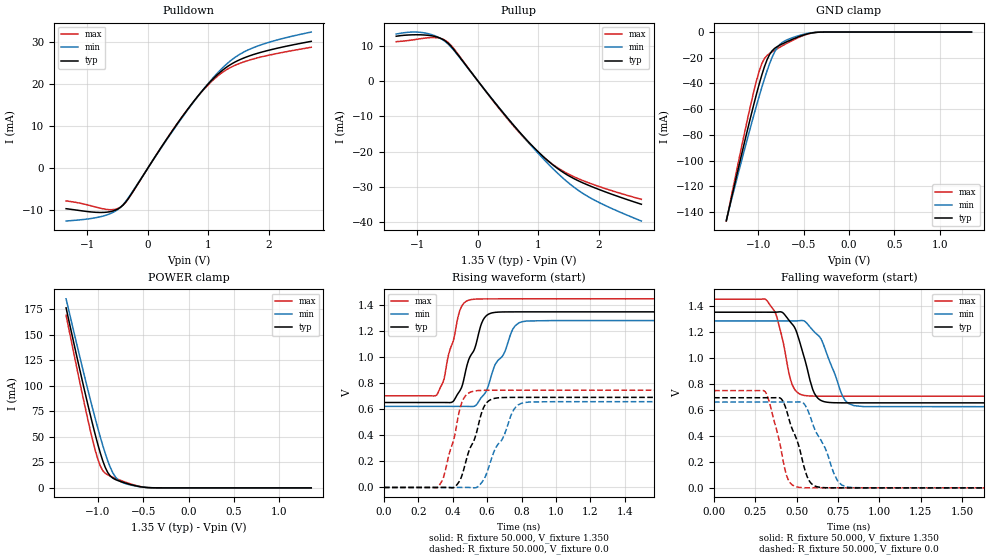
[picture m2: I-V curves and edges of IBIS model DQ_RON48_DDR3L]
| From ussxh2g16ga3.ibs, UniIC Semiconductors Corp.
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|   Model DQ_RON48_DDR3L
[Model] DQ_RON48_DDR3L
Model_type I/O
Vinl =  0.540V
Vinh =  0.810V
Vmeas =  0.675V
Rref =  50.000
Vref =  0.675V
C_comp   0.966pF   0.965pF   0.967pF
[Model Spec]
Vinh   0.810V   0.776V   0.860V
Vinl   0.540V   0.506V   0.590V
Vmeas   0.675V   0.641V   0.725V
Vref   0.675V   0.641V   0.725V
Rref   50.000   NA   NA
[Temperature Range]   25.000   95.000   -40.000
[Voltage Range]   1.350V   1.283V   1.450V
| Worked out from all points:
|   slope of the pulldown table from 0 to 0.203 V, typ, clamps not added: 44.6 ohm
|   slope of the pullup table from 0 to 0.203 V, typ, clamps not added: 45.5 ohm
|   GND clamp passes 1 mA (typ) near -0.43 V on its own axis
|   POWER clamp passes 1 mA (typ) near -0.52 V on its own axis
|   rising waveform, R_fixture 50.000, V_fixture 1.350: 20-80 % time 98.5ps typ, 130ps min, 76.3ps max; typ from 0.653 V to 1.35 V
|   rising waveform, R_fixture 50.000, V_fixture 0.0: 20-80 % time 99.3ps typ, 128ps min, 79.9ps max; typ from 0 V to 0.693 V
|   falling waveform, R_fixture 50.000, V_fixture 1.350: 20-80 % time 93.1ps typ, 118ps min, 75.9ps max; typ from 1.35 V to 0.653 V
|   falling waveform, R_fixture 50.000, V_fixture 0.0: 20-80 % time 102ps typ, 132ps min, 80.6ps max; typ from 0.693 V to 0 V
[Pulldown]
|Voltage   I(typ)   I(min)   I(max)
-1.35V    -9.661mA   -12.6mA    -7.804mA
-735mV    -10.55mA   -11.4mA    -9.699mA
-571mV    -10.19mA   -10.52mA   -9.878mA
-448mV    -9.296mA   -9.283mA   -9.257mA
-325mV    -7.31mA    -7.136mA   -7.371mA
249mV     5.557mA    5.434mA    5.606mA
618mV     13.25mA    13.09mA    13.27mA
905mV     18.55mA    18.56mA    18.43mA
1.151V    22.32mA    22.69mA    21.94mA
1.397V    24.97mA    25.97mA    24.24mA
1.684V    26.81mA    28.38mA    25.8mA
2.7V      30.25mA    32.47mA    28.84mA
[Pullup]
|Voltage   I(typ)   I(min)   I(max)
-1.35V    12.67mA    13.29mA    11.13mA
-908mV    13.04mA    13.68mA    12.07mA
-703mV    12.57mA    12.74mA    12.28mA
-539mV    11.33mA    11.14mA    11.5mA
-416mV    9.28mA     9.055mA    9.534mA
568mV     -12.09mA   -12.06mA   -12.31mA
855mV     -17.57mA   -17.78mA   -17.76mA
1.142V    -22.35mA   -23.11mA   -22.34mA
1.429V    -26.07mA   -27.83mA   -25.71mA
1.757V    -28.99mA   -32.05mA   -28.32mA
2.126V    -31.5mA    -35.4mA    -30.55mA
2.7V      -34.86mA   -39.6mA    -33.47mA
[GND_clamp]
|Voltage   I(typ)   I(min)   I(max)
-1.35V    -146.9mA   -146.3mA   -147.1mA
-1.126V   -78.8mA    -85.17mA   -70.77mA
-1.014V   -47.25mA   -56.31mA   -36.92mA
-958mV    -33.17mA   -42.77mA   -24.44mA
-930mV    -26.97mA   -36.36mA   -20.61mA
-874mV    -17.51mA   -24.69mA   -16.72mA
-818mV    -12.71mA   -15.46mA   -14.21mA
-762mV    -10.26mA   -9.751mA   -11.88mA
-706mV    -8.307mA   -6.907mA   -9.644mA
-538mV    -3.274mA   -2.499mA   -3.731mA
-398mV    -591.2uA   -439.3uA   -663.7uA
1.35V     0A         0A         0A
[POWER_clamp]
|Voltage   I(typ)   I(min)   I(max)
-1.35V    176.6mA    185.4mA    169.4mA
-1.198V   115.5mA    128.2mA    103.2mA
-1.114V   83.04mA    97.6mA     68.48mA
-1.058V   62.42mA    77.92mA    46.98mA
-1.002V   43.19mA    59.09mA    28.56mA
-946mV    26.54mA    41.57mA    16.92mA
-890mV    14.85mA    26.22mA    12.66mA
-834mV    9.439mA    14.55mA    10.39mA
-778mV    7.089mA    7.901mA    8.361mA
-638mV    3.198mA    2.764mA    3.815mA
-414mV    126.6uA    165.9uA    94.28uA
1.35V     0A         0A         0A
[Ramp]
| variable   typ   min   max
dV/dt_r   0.416/99.045p   0.396/0.128n   0.448/79.809p
dV/dt_f   0.418/92.332p   0.396/0.118n   0.447/75.961p
R_load = 50.000
[Rising Waveform]
R_fixture= 50.000
V_fixture= 1.350
V_fixture_min= 1.283
V_fixture_max= 1.450
|time   V(typ)   V(min)   V(max)
0s        653.2mV    623.3mV    704.3mV
306ps     653.2mV    623.3mV    710.5mV
348ps     653.2mV    623.3mV    827.3mV
406ps     667.2mV    623.3mV    1.141V
450ps     764.2mV    623.3mV    1.388V
507ps     1.02V      622.3mV    1.444V
598ps     1.323V     749.6mV    1.45V
751ps     1.35V      1.221V     1.45V
801ps     1.35V      1.274V     1.45V
3ns       1.35V      1.283V     1.45V
[Rising Waveform]
R_fixture= 50.000
V_fixture= 0.0
V_fixture_min= 0.0
V_fixture_max= 0.0
|time   V(typ)   V(min)   V(max)
0s        157.3nV    1.097uV    72.97nV
316ps     -25.78uV   3.116uV    5.409mV
348ps     124.4uV    5.006uV    85.1mV
425ps     22.16mV    -16.36uV   497.4mV
461ps     124.6mV    146.6uV    677.1mV
524ps     363.1mV    -3.017mV   740.9mV
605ps     661.7mV    138mV      747.2mV
754ps     692.5mV    596.5mV    747.5mV
816ps     692.6mV    652.5mV    747.5mV
3ns       692.6mV    659.5mV    747.5mV
[Falling Waveform]
R_fixture= 50.000
V_fixture= 1.350
V_fixture_min= 1.283
V_fixture_max= 1.450
|time   V(typ)   V(min)   V(max)
0s        1.35V      1.283V     1.45V
316ps     1.35V      1.283V     1.445V
375ps     1.35V      1.283V     1.332V
423ps     1.337V     1.283V     1.09V
476ps     1.253V     1.283V     784.4mV
546ps     1V         1.282V     710.4mV
628ps     689.3mV    1.174V     704.6mV
778ps     653.3mV    704.1mV    704.3mV
847ps     653.2mV    631.6mV    704.3mV
3ns       653.2mV    623.3mV    704.3mV
[Falling Waveform]
R_fixture= 50.000
V_fixture= 0.0
V_fixture_min= 0.0
V_fixture_max= 0.0
|time   V(typ)   V(min)   V(max)
0s        692.6mV    659.5mV    747.5mV
310ps     692.5mV    659.5mV    739.1mV
412ps     675.2mV    659.5mV    248.7mV
447ps     558.2mV    659.4mV    67.71mV
501ps     367.5mV    660mV      6.74mV
547ps     149.9mV    642.9mV    947.1uV
590ps     31.14mV    517.6mV    145.3uV
745ps     64.03uV    58.83mV    381.5nV
812ps     4.268uV    5.401mV    234.7nV
3ns       139.7nV    1.088uV    188.2nV
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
